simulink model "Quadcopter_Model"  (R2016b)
settings: Solver=VariableStepAuto  StartTime=0.0  StopTime=10.0  RelTol=1e-3

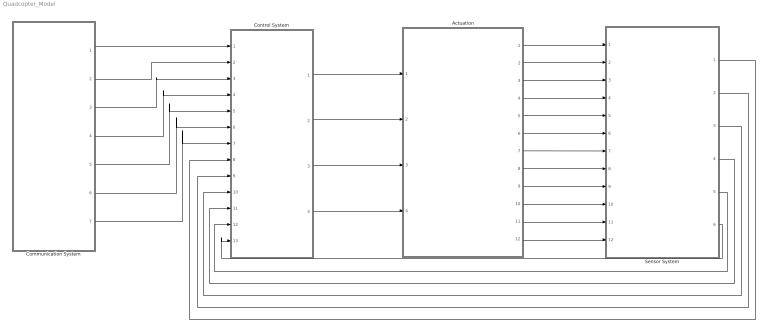
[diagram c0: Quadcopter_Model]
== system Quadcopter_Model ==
  Actuation : Subsystem
  Communication System : Subsystem
  Control System : Subsystem
  Sensor System : Subsystem
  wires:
  Control System/1(Rotor 0 Duty Cycle) -> Actuation/1(Rotor 0 Duty Cycle)
  Control System/2(Rotor 1 Duty Cycle) -> Actuation/2(Rotor 1 Duty Cycle)
  Control System/3(Rotor 2 Duty Cycle) -> Actuation/3(Rotor 2 Duty Cycle)
  Control System/4(Rotor 3 Duty Cycle) -> Actuation/4(Rotor 3 Duty Cycle)
  Actuation/1(Body frame linear velocity (u)) -> Sensor System/1(Body frame linear velocity (u))
  Actuation/2(Body frame linear velocity (v)) -> Sensor System/2(Body frame linear velocity (v))
  Actuation/3(Body frame linear velocity (w)) -> Sensor System/3(Body frame linear velocity (w))
  Actuation/4(Body frame angular velocity (p)) -> Sensor System/4(Body frame angular velocity (p))
  Actuation/5(Body frame angular velocity (q)) -> Sensor System/5(Body frame angular velocity (q))
  Actuation/6(Body frame angular velocity (r)) -> Sensor System/6(Body frame angular velocity (r))
  Actuation/7(Earth frame position (x)) -> Sensor System/7(Earth frame position (x))
  Actuation/8(Earth frame position (y)) -> Sensor System/8(Earth frame position (y))
  Actuation/9(Earth frame position (z)) -> Sensor System/9(Earth frame position (z))
  Actuation/10(Earth frame pitch (phi)) -> Sensor System/10(Earth frame pitch (phi))
  Actuation/11(Earth frame roll (theta)) -> Sensor System/11(Earth frame roll (theta))
  Actuation/12(Earth frame yaw (psi)) -> Sensor System/12(Earth frame yaw (psi))
  Sensor System/6(Yaw rate (psi dot)) -> Control System/13(Yaw rate (psi dot))
  Sensor System/5(Roll rate (theta dot)) -> Control System/12(Roll rate (theta dot))
  Sensor System/4(Pitch rate (phi dot)) -> Control System/11(Pitch rate (phi dot))
  Sensor System/3(Yaw (psi)) -> Control System/10(Yaw (psi))
  Sensor System/2(Roll (theta)) -> Control System/9(Roll (theta))
  Sensor System/1(Pitch (phi)) -> Control System/8(Pitch (phi))
  Communication System/1(x_position) -> Control System/1(x position)
  Communication System/2(y_position) -> Control System/2(y position)
  Communication System/3(z_position) -> Control System/3(z position)
  Communication System/4(x_setpoint) -> Control System/4(x setpoint)
  Communication System/5(y_setpoint) -> Control System/5(y setpoint)
  Communication System/6(z_setpoint) -> Control System/6(z setpoint)
  Communication System/7(yaw_setpoint) -> Control System/7("Yaw setpoint ")

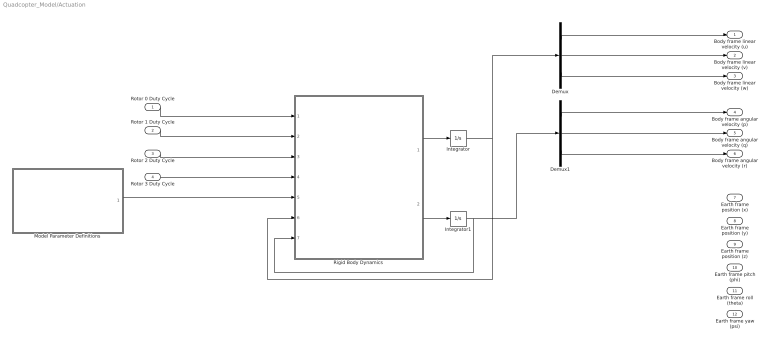
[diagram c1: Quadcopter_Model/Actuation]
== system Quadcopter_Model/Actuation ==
  Rotor 0 Duty Cycle : Inport
  Rotor 1 Duty Cycle : Inport  Port=2
  Rotor 2 Duty Cycle : Inport  Port=3
  Rotor 3 Duty Cycle : Inport  Port=4
  Demux : Demux  Outputs=3
  Demux1 : Demux  Outputs=3
  Integrator : Integrator
  Integrator1 : Integrator
  Model Parameter Definitions : MATLAB Function  TreatAsAtomicUnit=on
  Rigid Body Dynamics : MATLAB Function  TreatAsAtomicUnit=on
  Body frame linear velocity (u) : Outport
  Body frame linear velocity (v) : Outport  Port=2
  Body frame linear velocity (w) : Outport  Port=3
  Body frame angular velocity (p) : Outport  Port=4
  Body frame angular velocity (q) : Outport  Port=5
  Body frame angular velocity (r) : Outport  Port=6
  Earth frame position (x) : Outport  Port=7
  Earth frame position (y) : Outport  Port=8
  Earth frame position (z) : Outport  Port=9
  Earth frame pitch (phi) : Outport  Port=10
  Earth frame roll (theta) : Outport  Port=11
  Earth frame yaw (psi) : Outport  Port=12
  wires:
  Model Parameter Definitions/1(model_parameters) -> Rigid Body Dynamics/5(model_parameters)
  Rotor 3 Duty Cycle/1 -> Rigid Body Dynamics/4(rotor_3_duty_cycle)
  Rotor 2 Duty Cycle/1 -> Rigid Body Dynamics/3(rotor_2_duty_cycle)
  Rotor 0 Duty Cycle/1 -> Rigid Body Dynamics/1(rotor_0_duty_cycle)
  Rotor 1 Duty Cycle/1 -> Rigid Body Dynamics/2(rotor_1_duty_cycle)
  Integrator1/1 -> Demux1/1, Rigid Body Dynamics/7(b_v)
  Integrator/1 -> Rigid Body Dynamics/6(b_Omega), Demux/1
  Demux/1 -> Body frame linear velocity (u)/1
  Demux/2 -> Body frame linear velocity (v)/1
  Demux/3 -> Body frame linear velocity (w)/1
  Demux1/1 -> Body frame angular velocity (p)/1
  Demux1/2 -> Body frame angular velocity (q)/1
  Demux1/3 -> Body frame angular velocity (r)/1
  Rigid Body Dynamics/1(b_Omega_dot) -> Integrator/1
  Rigid Body Dynamics/2(b_v_dot) -> Integrator1/1

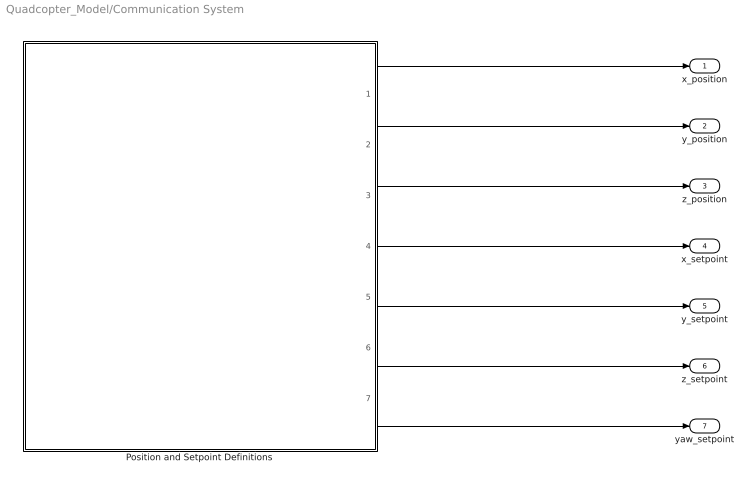
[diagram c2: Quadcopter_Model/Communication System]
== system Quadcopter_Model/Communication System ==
  Position and Setpoint Definitions : MATLAB Function  TreatAsAtomicUnit=on
  x_position : Outport
  y_position : Outport  Port=2
  z_position : Outport  Port=3
  x_setpoint : Outport  Port=4
  y_setpoint : Outport  Port=5
  z_setpoint : Outport  Port=6
  yaw_setpoint : Outport  Port=7
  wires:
  Position and Setpoint Definitions/7(yaw_setpoint) -> yaw_setpoint/1
  Position and Setpoint Definitions/6(z_setpoint) -> z_setpoint/1
  Position and Setpoint Definitions/5(y_setpoint) -> y_setpoint/1
  Position and Setpoint Definitions/4(x_setpoint) -> x_setpoint/1
  Position and Setpoint Definitions/3(z_position) -> z_position/1
  Position and Setpoint Definitions/2(y_position) -> y_position/1
  Position and Setpoint Definitions/1(x_position) -> x_position/1

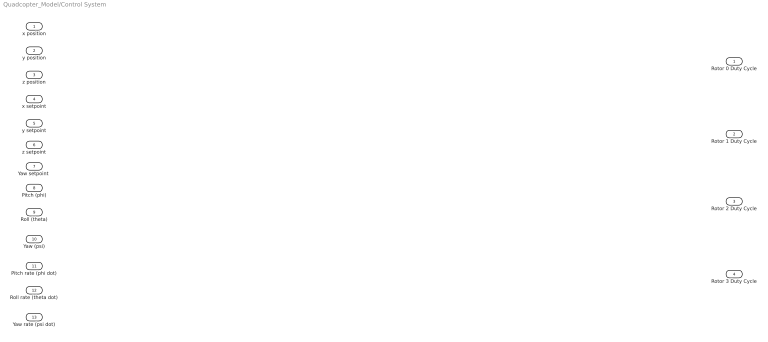
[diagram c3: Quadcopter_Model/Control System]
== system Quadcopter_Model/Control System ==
  x position : Inport
  y position : Inport  Port=2
  z position : Inport  Port=3
  x setpoint : Inport  Port=4
  y setpoint : Inport  Port=5
  z setpoint : Inport  Port=6
  "Yaw setpoint " : Inport  Port=7
  Pitch (phi) : Inport  Port=8
  Roll (theta) : Inport  Port=9
  Yaw (psi) : Inport  Port=10
  Pitch rate (phi dot) : Inport  Port=11
  Roll rate (theta dot) : Inport  Port=12
  Yaw rate (psi dot) : Inport  Port=13
  Rotor 0 Duty Cycle : Outport
  Rotor 1 Duty Cycle : Outport  Port=2
  Rotor 2 Duty Cycle : Outport  Port=3
  Rotor 3 Duty Cycle : Outport  Port=4

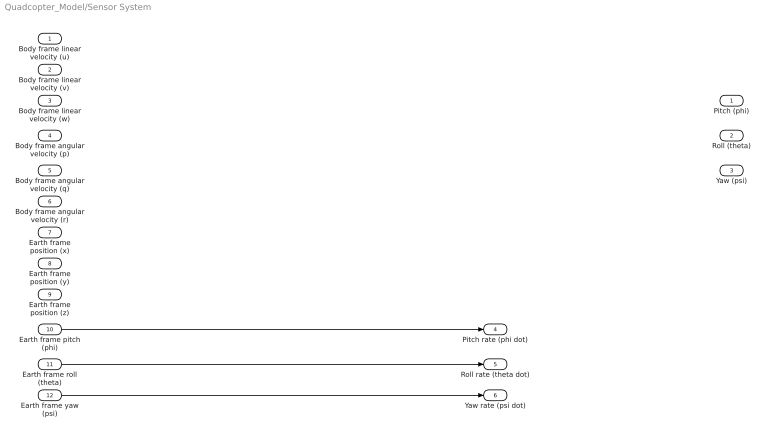
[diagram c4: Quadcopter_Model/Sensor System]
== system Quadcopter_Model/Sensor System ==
  Body frame linear velocity (u) : Inport
  Body frame linear velocity (v) : Inport  Port=2
  Body frame linear velocity (w) : Inport  Port=3
  Body frame angular velocity (p) : Inport  Port=4
  Body frame angular velocity (q) : Inport  Port=5
  Body frame angular velocity (r) : Inport  Port=6
  Earth frame position (x) : Inport  Port=7
  Earth frame position (y) : Inport  Port=8
  Earth frame position (z) : Inport  Port=9
  Earth frame pitch (phi) : Inport  Port=10
  Earth frame roll (theta) : Inport  Port=11
  Earth frame yaw (psi) : Inport  Port=12
  Pitch (phi) : Outport
  Roll (theta) : Outport  Port=2
  Yaw (psi) : Outport  Port=3
  Pitch rate (phi dot) : Outport  Port=4
  Roll rate (theta dot) : Outport  Port=5
  Yaw rate (psi dot) : Outport  Port=6
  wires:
  Earth frame pitch (phi)/1 -> Pitch rate (phi dot)/1
  Earth frame roll (theta)/1 -> Roll rate (theta dot)/1
  Earth frame yaw (psi)/1 -> Yaw rate (psi dot)/1

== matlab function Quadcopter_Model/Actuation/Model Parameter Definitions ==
function model_parameters = modelParameterDefinitions()
%This function defines and returns the quadcopter parameters used, as a
%struct.

    %Create an empty struct
    model_parameters = struct();
    
    %Fill model_parameters struct with the parameters of the quadcopter
    model_parameters.m = 1.19;            % Quadrotor + battery mass
    model_parameters.g = 9.81;            % Acceleration of gravity
    model_parameters.Jxx = 0.0218;        % Quadrotor and battery motor of inertia around bx (pitch)
    model_parameters.Jyy = 0.0277;        % Quadrotor and battery motor of inertia around by (roll)
    model_parameters.Jzz = 0.0332;        % Quadrotor and battery motor of inertia around bz (yaw)
    model_parameters.J = [Jxx, 0 , 0; ... % Quadrotor moment of inertia matrix
                           0, Jyy, 0; ...
                           0,  0, Jzz]; 
    model_parameters.Jreq = 0;            % Rotor and motor moment of inertia around axis of rotation
    model_parameters.Kt = 8.1558*10^-6;   % Rotor thrust constant
    model_parameters.Kh = 0;              % Rotor in-plane drag constant
    model_parameters.Kd = 0;              % Rotor drag constant
    model_parameters.rhx = 0.016;         % X-axis distance from center of mass to a rotor hub
    model_parameters.rhy = 0.016;         % Y-axis distance from center of mass to a rotor hub
    model_parameters.rhz = 0.003;         % Z-axis distance from center of mass to a rotor hub
    model_parameters.Rm = 0.2308;         % Motor resistance
    model_parameters.Kq = 96.3422;        % Motor torque constant
    model_parameters.Kv = 96.3422;        % Motor back emf constant
    model_parameters.If = 0.511;          % Motor internal friction current
    model_parameters.Pmin = 0.47;         % Minimum zybo output duty cycle command
    model_parameters.Pmax = 0.80;         % Maximum zybo output duty cycle command
    model_parameters.Tc = 0.01;           % Camera system sampling period
    model_parameters.tau_c = 0;           % Camera system total latency
    model_parameters.Vb = 11.1;           % Nominal battery voltage (V)
    
end

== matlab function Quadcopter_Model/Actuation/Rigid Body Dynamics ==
function [ b_Omega_dot, b_v_dot] = rigidBodyDynamics(rotor_0_duty_cycle, rotor_1_duty_cycle, rotor_2_duty_cycle, rotor_3_duty_cycle, model_parameters, b_Omega, b_v)

%Define vector from body frame origin to center of mass
br_oc = 0;

%Define 3x3 Identity Matrix
I = eye(3);

%Create gamma vectors
gamma_Ti = [0; 0; -1];
gamma_omega_03 = [0; 0; 1];  %Rotors 0 and 3 use this gamma_omega vector
gamma_omega_12 = [0; 0; -1]; %Rotors 1 and 2 use this gamma_omega vector

%Pull parameters from the model_parameters struct
Rm = model_parameters.Rm;
Kv = model_parameters.Kv;
Kq = model_parameters.Kq;
Kd = model_parameters.Kd;
Kt = model_parameters.Kt;
If = model_parameters.If;
Pmin = model_parameters.Pmin;
Pmax = model_parameters.Pmax;
Vb = model_parameters.Vb;
rhx = model_parameters.rhx;
rhy = model_parameters.rhy;
rhz = model_parameters.rhz;
Jreq = model_parameters.Jreq;
J = model_parameters.J;

%Create r_hi vector
rhi = [rhx; rhy; rhz];

%Define u_Pi for each of the rotors
u_P0 = (rotor_0_duty_cycle - Pmin) / (Pmax - Pmin);
u_P1 = (rotor_1_duty_cycle - Pmin) / (Pmax - Pmin);
u_P2 = (rotor_2_duty_cycle - Pmin) / (Pmax - Pmin);
u_P3 = (rotor_3_duty_cycle - Pmin) / (Pmax - Pmin);

%Define w_i numerator and denominators for each of the rotors
w_0_num = -1 + sqrt( 1 - 4*Rm*Kv*Kq*Kd*(Kv*Rm*If - Kv*u_P0*Vb) );
w_1_num = -1 + sqrt( 1 - 4*Rm*Kv*Kq*Kd*(Kv*Rm*If - Kv*u_P1*Vb) );
w_2_num = -1 + sqrt( 1 - 4*Rm*Kv*Kq*Kd*(Kv*Rm*If - Kv*u_P2*Vb) );
w_3_num = -1 + sqrt( 1 - 4*Rm*Kv*Kq*Kd*(Kv*Rm*If - Kv*u_P3*Vb) );
w_i_den = 2*Rm*Kv*Kq*Kd;

%Define w_i (angular velocity) for each of the rotors
w_0 = w_0_num / w_i_den;
w_1 = w_1_num / w_i_den;
w_2 = w_2_num / w_i_den;
w_3 = w_3_num / w_i_den;

%Define w_i_dot (angular acceleration) for each of the rotors
w_0_dot = diff(w_0);
w_1_dot = diff(w_1);
w_2_dot = diff(w_2);
w_3_dot = diff(w_3);

%Define the body force in the z-direction from each rotor
bF_0 = Kt * w_0 * w_0 * gamma_Ti;
bF_1 = Kt * w_1 * w_1 * gamma_Ti;
bF_2 = Kt * w_2 * w_2 * gamma_Ti;
bF_3 = Kt * w_3 * w_3 * gamma_Ti;

%Sum up the body forces in the z-direction from each vector to get the
%total body force in the z-direction
bF = bF_0 + bF_1 + bF_2 + bF_3;


bQ_d0 = -1 * Kd * w_0 * w_0 * gamma_omega_03;
bQ_d1 = -1 * Kd * w_1 * w_1 * gamma_omega_12;
bQ_d2 = -1 * Kd * w_2 * w_2 * gamma_omega_12;
bQ_d3 = -1 * Kd * w_3 * w_3 * gamma_omega_03;

bQ_d = bQ_d0 + bQ_d1 + bQ_d2 + bQ_d3;

bQ_Fi = cross( rhi, bF );

bQ_Li0 = -1 * Jreq * cross(bOmega, w_0 * gamma_omega_03) + w_0_dot * gamma_omega_03;
bQ_Li1 = -1 * Jreq * cross(bOmega, w_1 * gamma_omega_12) + w_1_dot * gamma_omega_12; 
bQ_Li2 = -1 * Jreq * cross(bOmega, w_2 * gamma_omega_12) + w_2_dot * gamma_omega_12; 
bQ_Li3 = -1 * Jreq * cross(bOmega, w_3 * gamma_omega_03) + w_3_dot * gamma_omega_03;

bQ_Li = bQ_Li0 + bQ_Li1 + bQ_Li2 + bQ_Li3;

bQ = bQ_d + bQ_Fi + bQ_Li;

b_v_dot = (m*I)^(-1) * (bF - cross(b_Omega, m*(b_v + cross(b_Omega, br_oc))));
b_Omega_dot = (J)^(-1) * (bQ - cross(b_Omega, J * b_Omega - cross(br_oc, bF)));

end

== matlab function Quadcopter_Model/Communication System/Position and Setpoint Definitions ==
function [x_position, y_position, z_position, x_setpoint,...
    y_setpoint, z_setpoint, yaw_setpoint]= positionAndSetpointDefinitions

x_position = 0;
y_position = 0;
z_position = 0;
x_setpoint = 0;
y_setpoint = 0;
z_setpoint = 0;
yaw_setpoint = 0;

end
